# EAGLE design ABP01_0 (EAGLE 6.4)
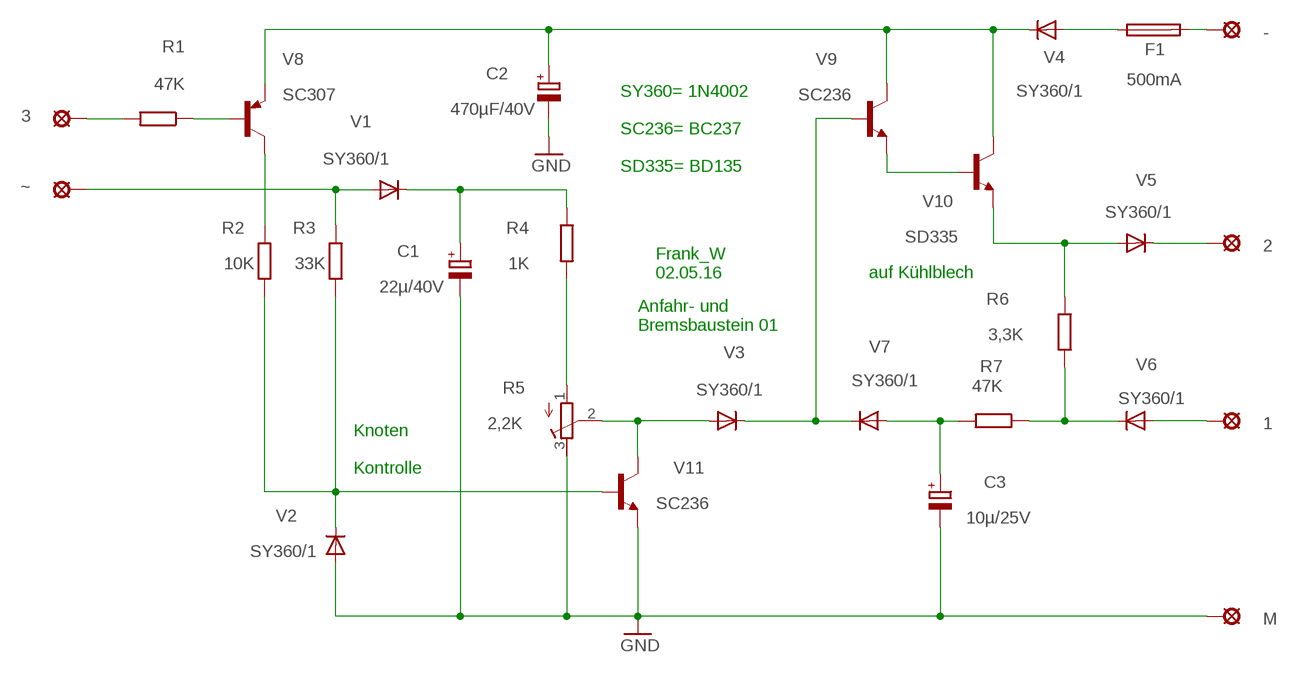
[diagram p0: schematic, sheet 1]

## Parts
1  LSP10  [LSP10]
2  LSP10  [LSP10]
3  LSP10  [LSP10]
-  LSP10  [LSP10]
C1  22µ/40V  CPOL-EUE5-5  [E5-5]
C2  470µF/40V  CPOL-EUE22-9AXIAL  [E22-9]
C3  10µ/25V  CPOL-EUE5-5  [E5-5]
F1  500mA  FUSEBLANK_5X20MM  [FUSE_HOLDER_5X20MM]
M  LSP10  [LSP10]
R1  47K  R-EU_0207/12  [0207/12]
R2  10K  R-EU_0207/12  [0207/12]
R3  33K  R-EU_0207/12  [0207/12]
R4  1K  R-EU_0207/12  [0207/12]
R5  2,2K  R-TRIMM64P  [RTRIM64P]
R6  3,3K  R-EU_0207/12  [0207/12]
R7  47K  R-EU_0207/12  [0207/12]
V1  SY360/1  1N4004  [DO41-10]
V2  SY360/1  1N4004  [DO41-10]
V3  SY360/1  1N4004  [DO41-10]
V4  SY360/1  1N4004  [DO41-10]
V5  SY360/1  1N4004  [DO41-10]
V6  SY360/1  1N4004  [DO41-10]
V7  SY360/1  1N4004  [DO41-10]
V8  SC307  BC327  [TO92]
V9  SC236  BC237  [TO92]
V10  SD335  BD139  [TO126]
V11  SC236  BC237  [TO92]
~  LSP10  [LSP10]

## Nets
GND: C1.- C2.- C3.- M.MP R5.3(E) V2.A V11.1(E)
N$1: -.MP F1.2
N$2: 3.MP R1.2
N$3: R1.1 V8.2(B)
N$4: R3.1 V1.A ~.MP
N$5: R2.1 V8.3(C)
N$6: C1.+ R4.1 V1.C
N$8: R4.2 R5.1(A)
N$9: F1.1 V4.A
N$10: R2.2 R3.2 V2.C V11.2(B)
N$11: R5.2(S) V3.A V11.3(C)
N$12: V3.C V7.C V9.2(B)
N$13: C3.+ R7.2 V7.A
N$14: R6.2 R7.1 V6.C
N$15: 1.MP V6.A
N$16: V9.1(E) V10.3(B)
N$17: R6.1 V5.A V10.1(E)
N$18: 2.MP V5.C
N$19: C2.+ V4.C V8.1(E) V9.3(C) V10.2(C)

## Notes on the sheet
- SY360= 1N4002
  
  SC236= BC237
  
  SD335= BD135
- Frank_W
  02.05.16
- auf Kühlblech
- Anfahr- und
  Bremsbaustein 01
- Knoten
  
  Kontrolle

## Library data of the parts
1-3 - M ~ = solpad:LSP10: SOLDER PAD
C1-C3 = rcl:CPOL-EU: POLARIZED CAPACITOR, European symbol
F1 = fuse:FUSE: Fuse; OC_FARNELL: unknown; OC_NEWARK: unknown
R1-R4 R6 R7 = rcl:R-EU_: RESISTOR, European symbol
R5 = rcl:R-TRIMM: Trimm resistor
V1-V7 = diode:1N4004: DIODE
V8 = transistor-pnp:BC327: PNP Transistor
V9 V11 = transistor-neu-to92:BC237: NPN TRANSISTOR
V10 = transistor:BD139: NPN TRANSISTOR

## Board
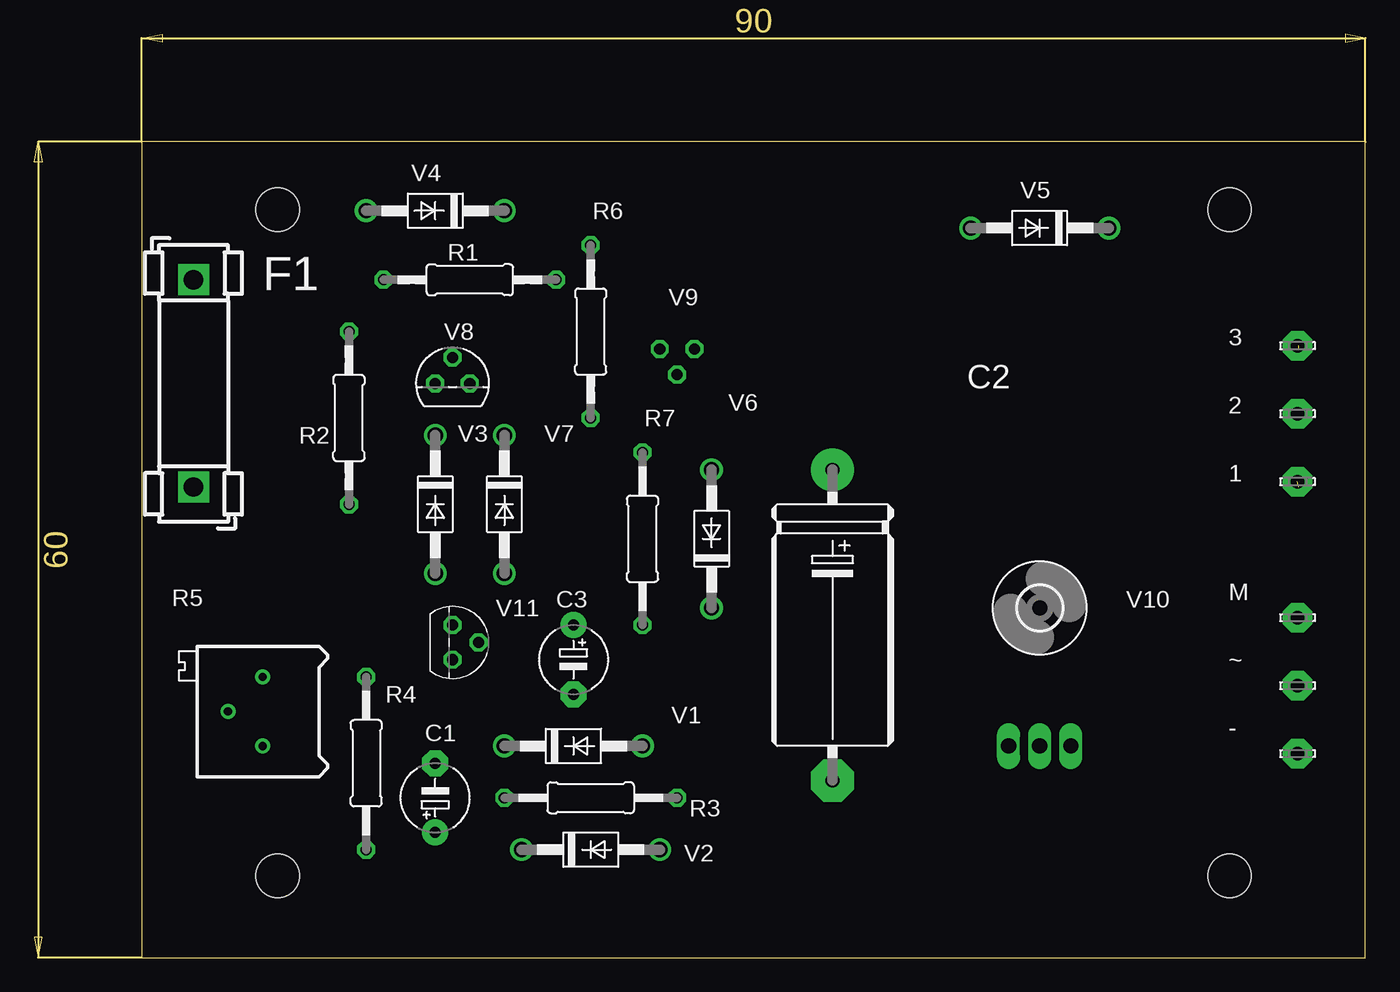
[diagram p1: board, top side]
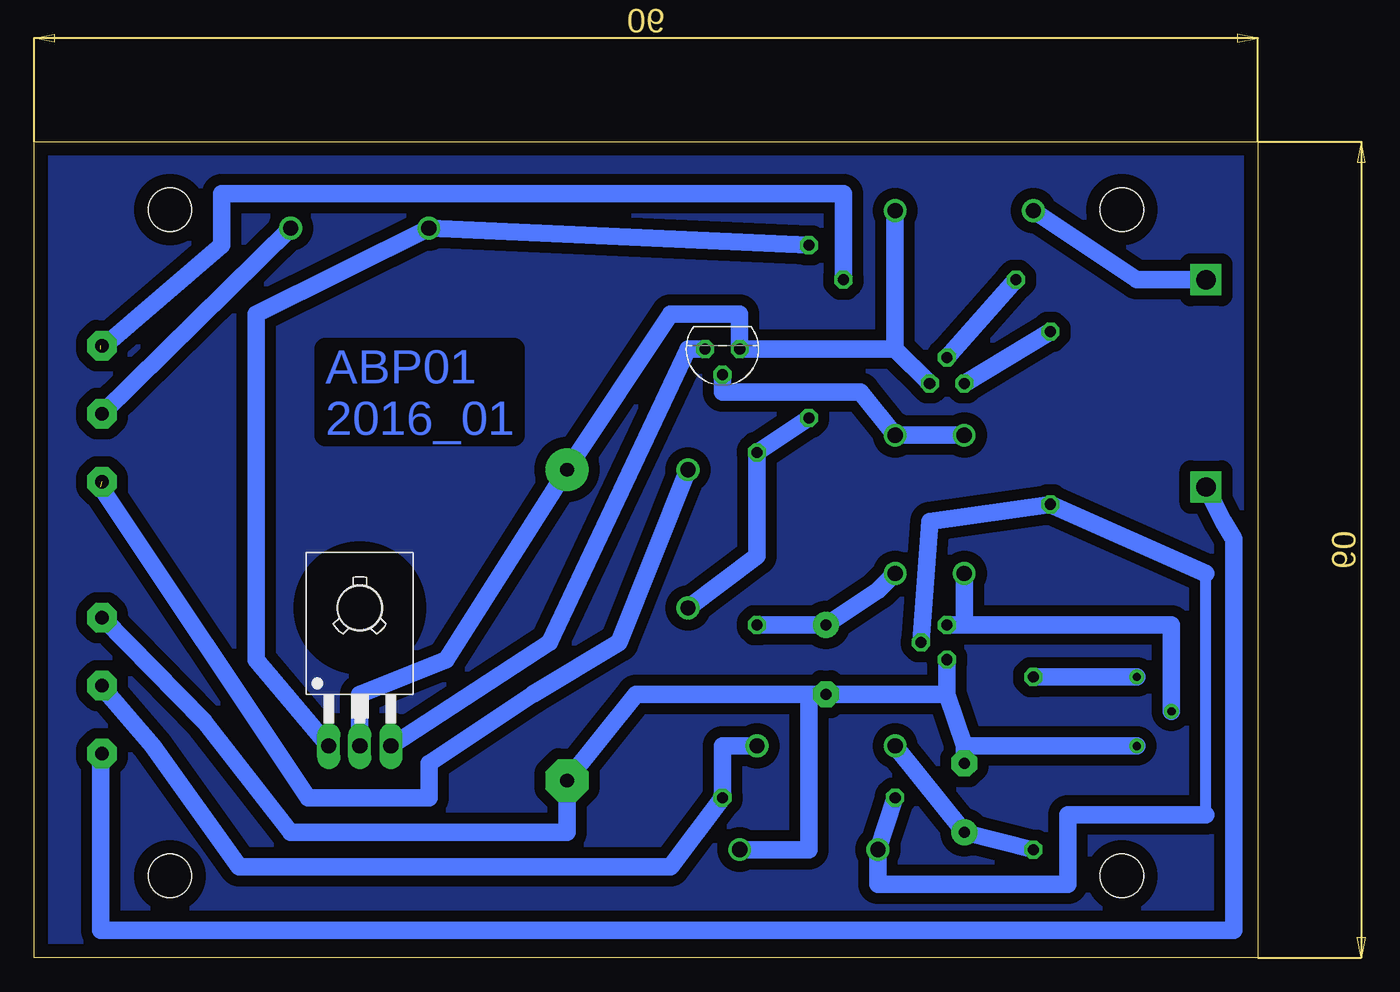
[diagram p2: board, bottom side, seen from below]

Size 97.92 x 67.93 mm. Coordinates in mm from the lower left corner, seen from the top.
Outline: 7.92,0 97.92,0 97.92,60 7.92,60 7.92,0
Copper layers (1*16): Top 0.035mm / dielectric 1.5mm / Bottom 0.035mm
Design rules "default *": minimum track width 20mil, minimum drill 24mil, track to track 8mil, track to pad 8mil, pad to pad 8mil, via to via 8mil, smd to smd 8mil, copper to edge 40mil, drill to drill 8mil, minimum pad ring 10mil, minimum via ring 8mil, stop-mask expansion 4mil, vias tented up to drill 0mil, thermal gap 20mil
Holes 3.2 mm at 87.92,55 87.92,6 17.92,6 17.92,55

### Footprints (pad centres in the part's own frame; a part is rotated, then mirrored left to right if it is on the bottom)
LSP10 = drill 1.016 pad 2.159 octagon: MP 0,0
E5-5 = drill 0.813 pad 1.905: + -2.54,0 | drill 0.813 pad 1.905 octagon: - 2.54,0
E22-9 = drill 1.016 pad 3.15: + -11.43,0 | drill 1.016 pad 3.15 octagon: - 11.43,0
FUSE_HOLDER_5X20MM = drill 1.422 pad 2.286 square: 1 0,0; 2 15.24,0
0207/12 = drill 0.813 octagon: 1 -6.35,0; 2 6.35,0
RTRIM64P = drill 0.61: 1 0,-2.54; 2 2.54,0; 3 0,2.54
3,2 = hole 3.2: 0,0
DO41-10 = drill 1.118: A 5.08,0; C -5.08,0
TO92 = drill 0.813 octagon: 1 1.27,0; 2 0,1.905; 3 -1.27,0
TO126 = drill 1.118 long: 1 -2.286,-5.08; 2 0,-5.08; 3 2.286,-5.08 | hole 3.302: 0,5.08

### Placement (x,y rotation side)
1  92.92,35 0 top
2  92.92,40 0 top
3  92.92,45 0 top
-  92.92,15 0 top
C1  29.51,11.75 90 top
C2  58.72,24.45 270 top
C3  39.67,21.91 270 top
F1  11.73,49.85 270 top
M  92.92,25 0 top
R1  32.05,49.85 0 top
R2  23.16,39.69 270 top
R3  40.94,11.75 180 top
R4  24.43,14.29 90 top
R5  16.81,18.1 180 top
R6  40.94,46.04 270 top
R7  44.75,30.8 270 top
U$1  [3,2]  73.96,25.72 0 top
V1  39.67,15.56 0 top
V2  40.94,7.94 0 top
V3  29.51,33.34 270 top
V4  29.51,54.93 180 top
V5  73.96,53.66 180 top
V6  49.83,30.8 90 top
V7  34.59,33.34 270 top
V8  30.78,42.23 0 top
V9  47.29,44.77 180 bottom
V10  73.96,20.64 0 bottom
V11  30.78,23.18 270 top
~  92.92,20 0 top

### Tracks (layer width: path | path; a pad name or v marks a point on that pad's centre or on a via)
GND
  Bottom 1.27: 29.51,15.56 R5.3 | C1.- 29.51,15.56 | V11.1 30.78,19.37 | 30.78,19.37 29.51,15.56 | 30.78,19.37 C3.- 40.94,19.37 | M.MP 85.39,17.38 79.04,9.21 58.72,9.21 C2.- 53.64,19.37 40.94,19.37 | V2.A 40.94,7.94 40.94,19.37
N$1
  Bottom 1.27: -.MP 93.01,15 93.01,2 9.67,2 9.67,30.8 10.46,32.07 F1.2
N$2  (1 unrouted)
  Bottom 1.27: 3.MP 93.01,45 | 93.01,44.77 84.12,52.39 84.12,56.2 38.4,56.2 R1.2
N$3
  Bottom 1.27: V8.2 R1.1
N$4
  Bottom 1.27: ~.MP 93.01,20 89.2,15.56 82.85,6.67 51.1,6.67 R3.1 47.29,15.56 V1.A
N$5
  Bottom 1.27: V8.3 R2.1
N$6
  Bottom 1.27: R4.1 C1.+ V1.C
N$7
  pour Bottom (isolate 0.813): 7.92,60.01 98.09,60.01 98.09,0.32 7.92,0.32
N$8
  Bottom 1.27: R4.2 R5.1
N$9
  Bottom 1.27: F1.1 16.81,49.85 V4.A
N$10
  Bottom 0.813: 11.73,10.48 11.73,28.26
  Bottom 1.27: V11.2 32.05,32.07 R2.2 11.73,28.26 | R3.2 V2.C 35.86,5.4 21.89,5.4 21.89,10.48 11.73,10.48
N$11
  Bottom 1.27: R5.2 14.27,24.45 29.51,24.45 | 29.51,24.45 V11.3 | V3.A 29.51,24.45
N$12
  Bottom 1.27: V9.2 47.29,41.59 37.13,41.59 V7.C V3.C
N$13
  Bottom 1.27: R7.2 C3.+ 35.86,26.99 V7.A
N$14
  Bottom 1.27: V6.C 44.75,29.53 R7.1 R6.2
N$15  (1 unrouted)
  Bottom 1.27: 93.01,34.61 77.77,11.75 68.88,11.75 68.88,14.29 61.26,19.37 54.91,23.18 V6.A
N$16
  Bottom 1.27: V10.3 59.99,23.18 49.83,44.77 V9.1
N$17
  Bottom 1.27: R6.1 V5.A 81.58,47.31 81.58,21.91 V10.1
N$18
  Bottom 1.27: 2.MP V5.C
N$19
  Bottom 1.27: V10.2 73.96,19.37 67.61,21.91 C2.+ 51.1,47.31 46.02,47.31 V9.3 34.59,44.77 | 34.59,44.77 V4.C | V8.1 34.59,44.77

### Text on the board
Bottom: ABP01 / 2016_01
